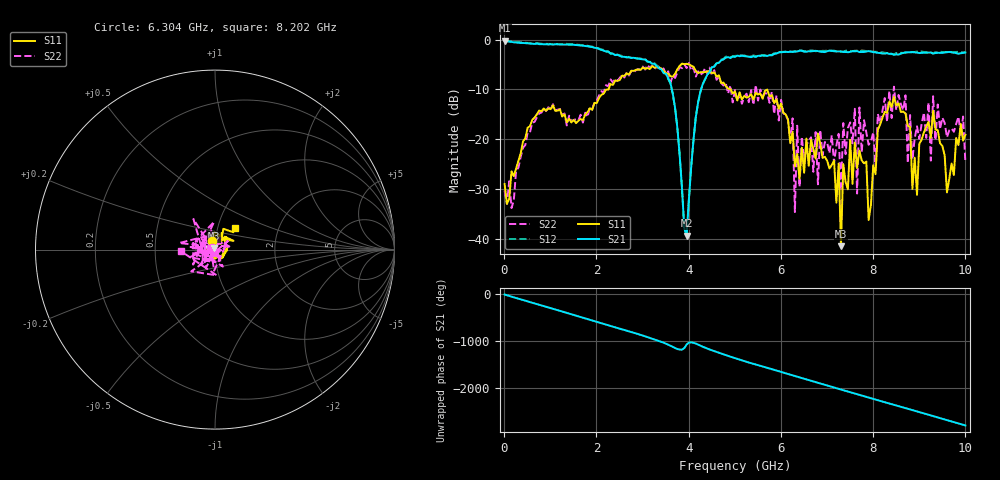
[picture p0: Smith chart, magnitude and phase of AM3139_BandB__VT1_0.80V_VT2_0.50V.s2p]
! Date/Time: Tue, Nov 13, 2018 4:59 PM
! Network Analyzer: Agilent Technologies E8364B Rev: A.07.50.67
! Sweep from 0.010 to 10.000 GHz, 201 Points, Sweep Type: LIN
! Power Supply: 0.800 V, 0.000 A
# Hz S DB R 50
!freq MagS11 AngS11 MagS21 AngS21 MagS12 AngS12 MagS22 AngS22
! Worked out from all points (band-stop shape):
!   201 points, 10 MHz to 10 GHz, reference 50 ohm
!   highest |S21| = -0.17 dB at 10 MHz (marker M1); lowest = -39.4 dB at 3.956 GHz (marker M2)
!   |S21| within 3 dB of the highest: start of sweep to 2.488 GHz; 5.734 GHz to end of sweep
!   lowest |S11| = -41.5 dB at 7.303 GHz (marker M3), VSWR 1.02, Z = 49.5 + j0.682 ohm
!   |S11| at or under -10 dB: start of sweep to 2.26 GHz; 4.91 GHz to end of sweep
!   |S22| runs from -34.6 to -4.7 dB; largest |S21 - S12| = 0.032
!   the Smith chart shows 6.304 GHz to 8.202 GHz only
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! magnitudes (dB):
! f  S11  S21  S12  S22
! 10 MHz  -29.0  -0.2  -0.1  -30.3
! 1.708 GHz  -16.1  -1.2  -1.1  -16.7
! 3.357 GHz  -5.6  -5.7  -5.5  -5.6
! 3.956 GHz  -4.8  -39.4  -39.0  -5.7
! 4.256 GHz  -6.5  -10.4  -10.5  -7.0
! 5.005 GHz  -10.4  -3.4  -3.3  -10.1
! 6.254 GHz  -18.5  -2.4  -2.4  -15.8
! 6.304 GHz  -25.5  -2.4  -2.3  -34.6
! 6.703 GHz  -22.0  -2.3  -2.2  -26.5
! 7.253 GHz  -24.9  -2.3  -2.4  -18.9
! 7.303 GHz  -41.5  -2.4  -2.4  -30.5
! 7.502 GHz  -20.1  -2.4  -2.2  -16.6
! 7.602 GHz  -20.7  -2.3  -2.2  -13.9
! 7.652 GHz  -25.8  -2.3  -2.2  -30.9
! 7.702 GHz  -22.3  -2.5  -2.4  -13.6
! 7.902 GHz  -36.2  -2.3  -2.3  -21.1
! 8.352 GHz  -12.4  -2.8  -2.9  -10.3
! 8.951 GHz  -31.2  -2.6  -2.4  -17.4
! 9.251 GHz  -19.7  -2.6  -2.6  -24.3
! 9.301 GHz  -14.3  -2.8  -2.7  -11.4
! 9.6 GHz  -30.7  -2.5  -2.5  -19.6
! 10 GHz  -19.1  -2.6  -2.5  -24.7
